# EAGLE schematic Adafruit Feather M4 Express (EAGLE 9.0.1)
COMPANY: ADAFRUIT INDUSTRIES; DRAWN: KTOWN; REV: B
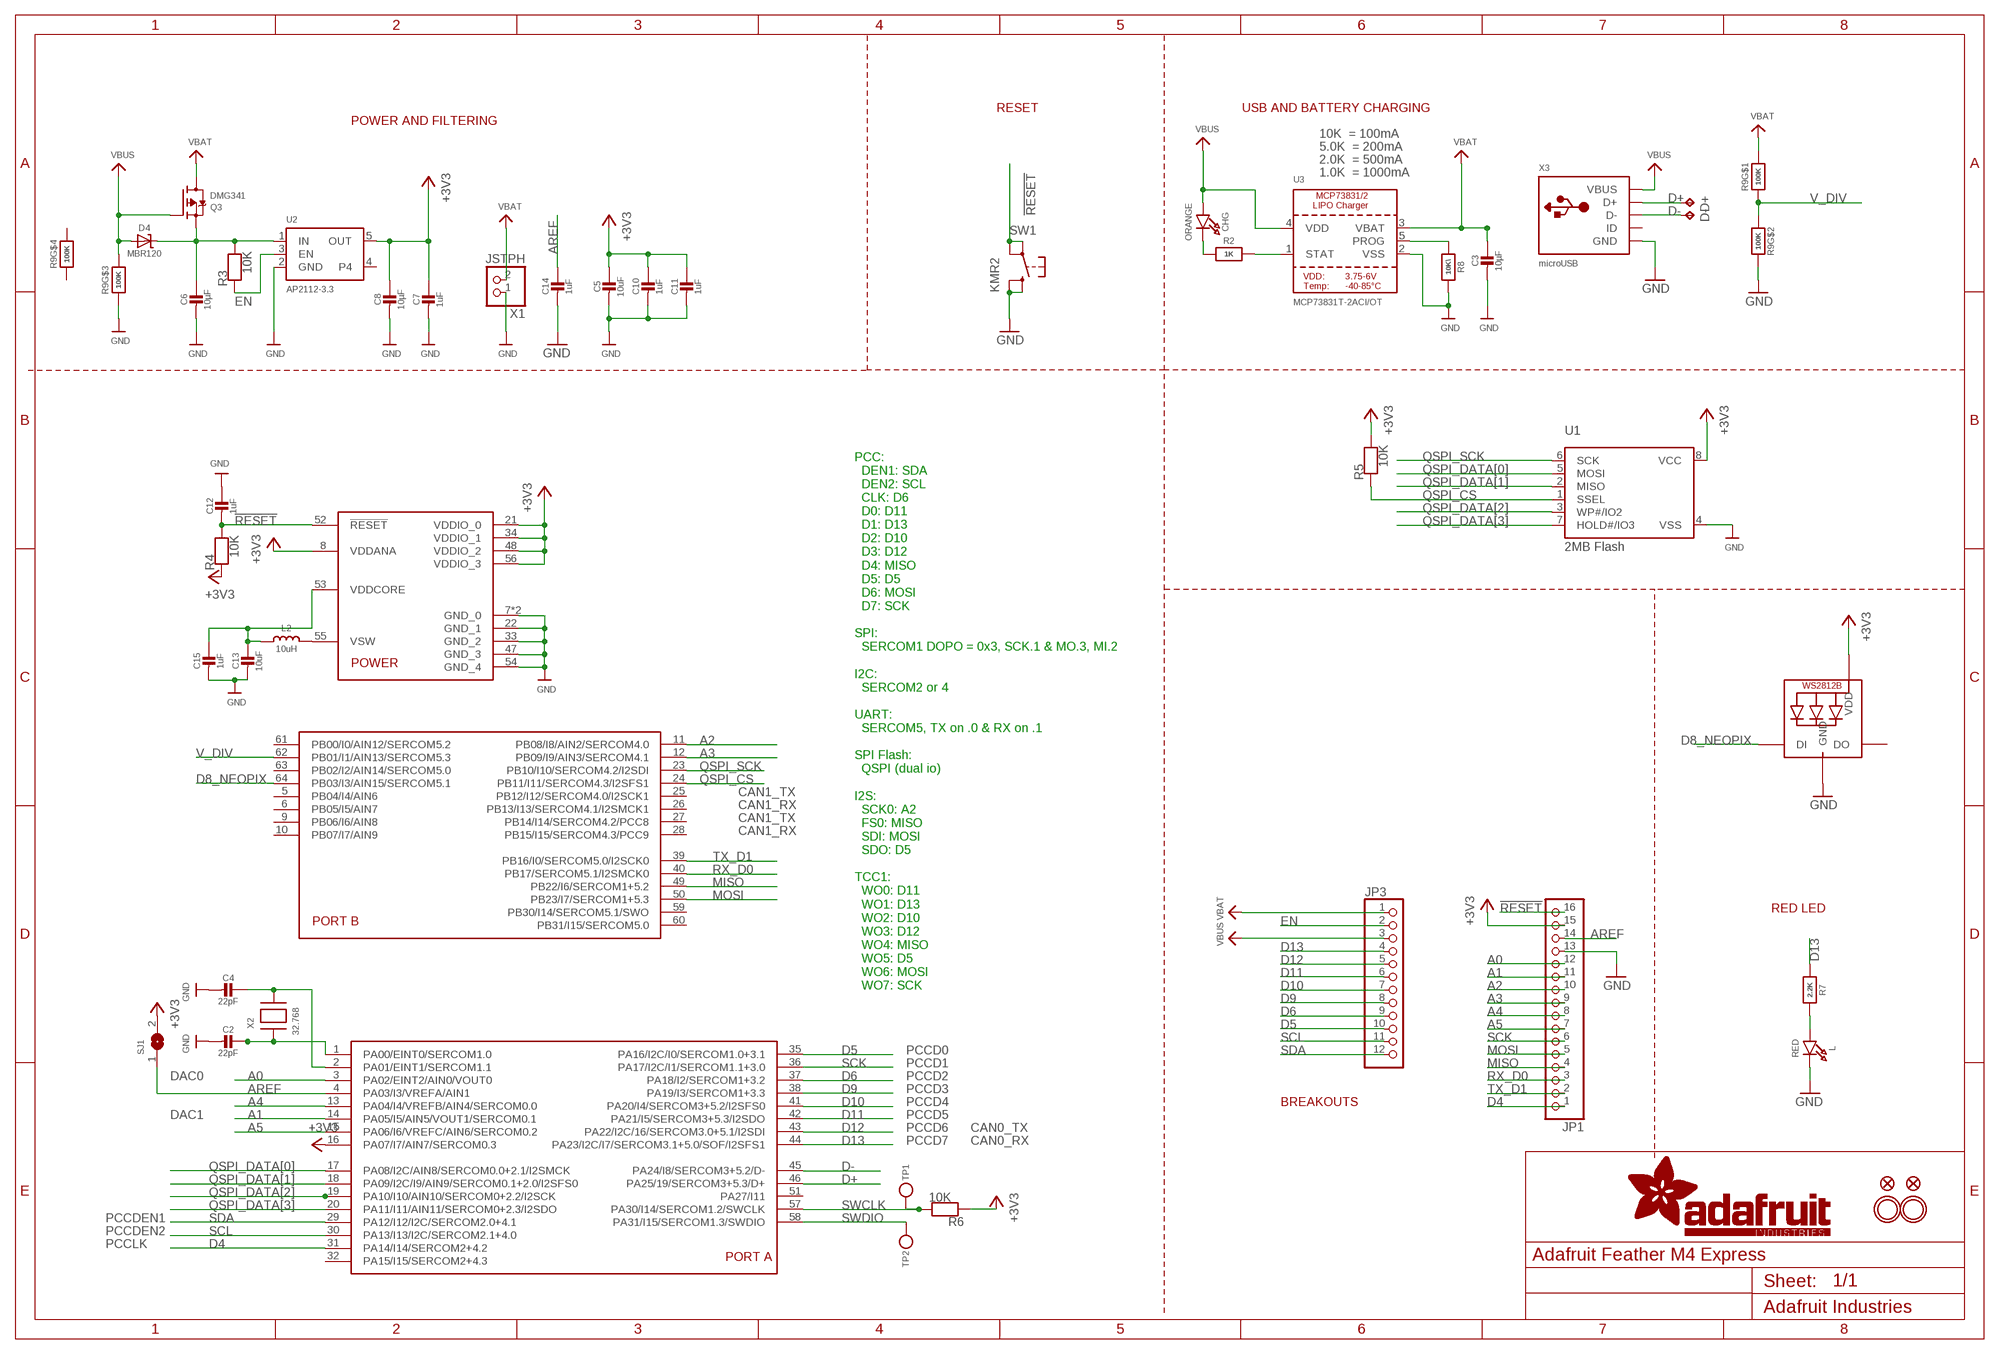
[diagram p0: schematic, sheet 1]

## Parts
C2  22pF  CAP_CERAMIC0603_NO  [0603-NO]
C3  10µF  CAP_CERAMIC0805-NOOUTLINE  [0805-NO]
C4  22pF  CAP_CERAMIC0603_NO  [0603-NO]
C5  10uF  CAP_CERAMIC0805-NOOUTLINE  [0805-NO]
C6  10µF  CAP_CERAMIC0805-NOOUTLINE  [0805-NO]
C7  1uF  CAP_CERAMIC0603_NO  [0603-NO]
C8  10µF  CAP_CERAMIC0805-NOOUTLINE  [0805-NO]
C10  1uF  CAP_CERAMIC0603_NO  [0603-NO]
C11  1uF  CAP_CERAMIC0603_NO  [0603-NO]
C12  1uF  CAP_CERAMIC0603_NO  [0603-NO]
C13  10uF  CAP_CERAMIC0805-NOOUTLINE  [0805-NO]
C14  1uF  CAP_CERAMIC0603_NO  [0603-NO]
C15  1uF  CAP_CERAMIC0603_NO  [0603-NO]
CHG  ORANGE  LED0805_NOOUTLINE  [CHIPLED_0805_NOOUTLINE]
D4  MBR120  DIODE-SCHOTTKYSOD-123  [SOD-123]
D+  TPB1,27  [B1,27]
D-  TPB1,27  [B1,27]
JP1  HEADER-1X16ROUND  [1X16_ROUND]
JP3  HEADER-1X12  [1X12_ROUND]
L  RED  LED0805_NOOUTLINE  [CHIPLED_0805_NOOUTLINE]
L2  10uH  INDUCTOR  [INDUCTOR_1007]
LED1  WS2812B3535  [LED3535]
Q3  DMG341  MOSFET-P  [SOT23-R]
R2  1K  RESISTOR_0603_NOOUT  [0603-NO]
R3  10K  RESISTOR_0603_NOOUT  [0603-NO]
R4  10K  RESISTOR_0603_NOOUT  [0603-NO]
R5  10K  RESISTOR_0603_NOOUT  [0603-NO]
R6  10K  RESISTOR_0603_NOOUT  [0603-NO]
R7  2.2K  RESISTOR_0603_NOOUT  [0603-NO]
R8  10K\  RESISTOR_0603_NOOUT  [0603-NO]
R9  100K  RESISTOR_4PACK_NO  [RESPACK_4X0603_NO]
SJ1  SOLDERJUMPERCLOSED  [SOLDERJUMPER_CLOSEDWIRE]
SW1  KMR2  SWITCH_TACT_SMT4.6X2.8  [BTN_KMR2_4.6X2.8]
TP1  TESTPOINTROUND1.5MM  [TESTPOINT_ROUND_1.5MM]
TP2  TESTPOINTROUND1.5MM  [TESTPOINT_ROUND_1.5MM]
U1  2MB Flash  SPIFLASH_8PINUX  [USON8]
U2  AP2112-3.3  VREG_SOT23-5  [SOT23-5]
U3  MCP73831T-2ACI/OT  MCP73831/2  [SOT23-5]
U$14  ATSAMD51J  [PQFN64-1]
U$31  MOUNTINGHOLE2.5  [MOUNTINGHOLE_2.5_PLATED]
U$32  MOUNTINGHOLE2.5  [MOUNTINGHOLE_2.5_PLATED]
U$34  FIDUCIAL_1MM  [FIDUCIAL_1MM]
U$35  FIDUCIAL_1MM  [FIDUCIAL_1MM]
X1  JSTPH  CON_JST_PH_2PIN  [JSTPH2]
X2  32.768  XTAL-3.2X1.5  [XTAL3215]
X3  microUSB  USB_MICRO_20329_V2  [4UCONN_20329_V2]

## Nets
!RESET: C12.2 JP1.16 R4.2 SW1.A'(P1) SW1.A(P) U$14.52(!RESET)
+3V3 [power]: C5.1 C7.1 C8.1 C10.1 C11.1 JP1.15 LED1.2(VDD) R4.1 R5.2 R6.1 SJ1.2 U1.8(VCC) U2.5(OUT) U$14.8(VDDANA) U$14.16(PA07/I7/AIN7/SERCOM0.3) U$14.21(VDDIO_0) U$14.34(VDDIO_1) U$14.48(VDDIO_2) U$14.56(VDDIO_3)
A0: JP1.12 U$14.3(PA02/EINT2/AIN0/VOUT0)
A1: JP1.11 U$14.14(PA05/I5/AIN5/VOUT1/SERCOM0.1)
A2: JP1.10 U$14.11(PB08/I8/AIN2/SERCOM4.0)
A3: JP1.9 U$14.12(PB09/I9/AIN3/SERCOM4.1)
A4: JP1.8 U$14.13(PA04/I4/VREFB/AIN4/SERCOM0.0)
A5: JP1.7 U$14.15(PA06/I6/VREFC/AIN6/SERCOM0.2)
AREF: C14.1 JP1.14 SJ1.1 U$14.4(PA03/I3/VREFA/AIN1)
D4: JP1.1 U$14.31(PA14/I14/SERCOM2+4.2)
D5: JP3.10 U$14.35(PA16/I2C/I0/SERCOM1.0+3.1)
D6: JP3.9 U$14.37(PA18/I2/SERCOM1+3.2)
D8_NEOPIX: LED1.1(DI) U$14.64(PB03/I3/AIN15/SERCOM5.1)
D9: JP3.8 U$14.38(PA19/I3/SERCOM1+3.3)
D10: JP3.7 U$14.41(PA20/I4/SERCOM3+5.2/I2SFS0)
D11: JP3.6 U$14.42(PA21/I5/SERCOM3+5.3/I2SDO)
D12: JP3.5 U$14.43(PA22/I2C/16/SERCOM3.0+5.1/I2SDI)
D13: JP3.4 R7.1 U$14.44(PA23/I2C/I7/SERCOM3.1+5.0/SOF/I2SFS1)
D+: D+.TP U$14.46(PA25/19/SERCOM3+5.3/D+) X3.D+
D-: D-.TP U$14.45(PA24/I8/SERCOM3+5.2/D-) X3.D-
EN: JP3.2 R3.1 U2.3(EN)
GND [gnd]: C2.2 C3.2 C4.2 C5.2 C6.2 C7.2 C8.2 C10.2 C11.2 C12.1 C13.2 C14.2 C15.2 JP1.13 L.C LED1.4(GND) R8.2 R9.3 R9.7 SW1.B'(S1) SW1.B(S) U1.4(VSS) U2.2(GND) U3.2(VSS) U$14.7(GND_0) U$14.22(GND_1) U$14.33(GND_2) U$14.47(GND_3) U$14.54(GND_4) U$14.EXP(GND_0) X1.1 X3.BASE@1(GND) X3.BASE@2(GND) X3.GND X3.SPRT@1(GND) X3.SPRT@2(GND) X3.SPRT@3(GND) X3.SPRT@4(GND)
MISO: JP1.4 U$14.49(PB22/I6/SERCOM1+5.2)
MOSI: JP1.5 U$14.50(PB23/I7/SERCOM1+5.3)
N$1: CHG.C R2.1
N$2: L.A R7.2
N$3: R2.2 U3.1(STAT)
N$4: R8.1 U3.5(PROG)
N$5: C2.1 U$14.1(PA00/EINT0/SERCOM1.0) X2.P$1
N$7: C4.1 U$14.2(PA01/EINT1/SERCOM1.1) X2.P$2
N$11: L2.P$2 U$14.55(VSW)
QSPI_CS: R5.1 U1.1(SSEL) U$14.24(PB11/I11/SERCOM4.3/I2SFS1)
QSPI_DATA[0]: U1.5(MOSI) U$14.17(PA08/I2C/AIN8/SERCOM0.0+2.1/I2SMCK)
QSPI_DATA[1]: U1.2(MISO) U$14.18(PA09/I2C/I9/AIN9/SERCOM0.1+2.0/I2SFS0)
QSPI_DATA[2]: U1.3(WP#/IO2) U$14.19(PA10/I10/AIN10/SERCOM0+2.2/I2SCK)
QSPI_DATA[3]: U1.7(HOLD#/IO3) U$14.20(PA11/I11/AIN11/SERCOM0+2.3/I2SDO)
QSPI_SCK: U1.6(SCK) U$14.23(PB10/I10/SERCOM4.2/I2SDI)
RX_D0: JP1.3 U$14.40(PB17/SERCOM5.1/I2SMCK0)
SCK: JP1.6 U$14.36(PA17/I2C/I1/SERCOM1.1+3.0)
SCL: JP3.11 U$14.30(PA13/I13/I2C/SERCOM2.1+4.0)
SDA: JP3.12 U$14.29(PA12/I12/I2C/SERCOM2.0+4.1)
SWCLK: R6.2 TP1.P$1 U$14.57(PA30/I14/SERCOM1.2/SWCLK)
SWDIO: TP2.P$1 U$14.58(PA31/I15/SERCOM1.3/SWDIO)
TX_D1: JP1.2 U$14.39(PB16/I0/SERCOM5.0/I2SCK0)
V_DIV: R9.1 R9.2 U$14.62(PB01/I1/AIN13/SERCOM5.3)
VBAT [power]: C3.1 JP3.1 Q3.3(D) R9.8 U3.3(VBAT) X1.2
VBUS [power]: CHG.A D4.A JP3.3 Q3.1(G) R9.6 U3.4(VDD) X3.VBUS
VDDCORE1: C13.1 C15.1 L2.P$1 U$14.53(VDDCORE)
VHI: C6.1 D4.C Q3.2(S) R3.2 U2.1(IN)
Unconnected: LED1.3(DO) R9.4 R9.5 U2.4 U$14.5(PB04/I4/AIN6) U$14.6(PB05/I5/AIN7) U$14.9(PB06/I6/AIN8) U$14.10(PB07/I7/AIN9) U$14.25(PB12/I12/SERCOM4.0/I2SCK1) U$14.26(PB13/I13/SERCOM4.1/I2SMCK1) U$14.27(PB14/I14/SERCOM4.2/PCC8) U$14.28(PB15/I15/SERCOM4.3/PCC9) U$14.32(PA15/I15/SERCOM2+4.3) U$14.51(PA27/I11) U$14.59(PB30/I14/SERCOM5.1/SWO) U$14.60(PB31/I15/SERCOM5.0) U$14.61(PB00/I0/AIN12/SERCOM5.2) U$14.63(PB02/I2/AIN14/SERCOM5.0) X3.ID

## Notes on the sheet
- RESET | USB AND BATTERY CHARGING
- POWER AND FILTERING
- 10K  = 100mA
- 5.0K  = 200mA
- 2.0K  = 500mA
- 1.0K  = 1000mA
- CAN1_TX
- CAN1_RX
- CAN1_TX
- CAN1_RX
- RED LED
- PCC:
    DEN1: SDA
    DEN2: SCL
    CLK: D6
    D0: D11
    D1: D13
    D2: D10
    D3: D12
    D4: MISO
    D5: D5
    D6: MOSI
    D7: SCK
  
  SPI:
    SERCOM1 DOPO = 0x3, SCK.1 & MO.3, MI.2
  
  I2C:
    SERCOM2 or 4
  
  UART:
    SERCOM5, TX on .0 & RX on .1
  
  SPI Flash:
    QSPI (dual io)
  
  I2S:
    SCK0: A2
    FS0: MISO
    SDI: MOSI
    SDO: D5
  
  TCC1:
    WO0: D11
    WO1: D13
    WO2: D10
    WO3: D12
    WO4: MISO
    WO5: D5
    WO6: MOSI
    WO7: SCK
- PCCD0
- PCCD1
- DAC0 | PCCD2
- PCCD3
- PCCD4 | BREAKOUTS
- DAC1 | PCCD5
- PCCD6 | CAN0_TX
- PCCD7 | CAN0_RX
- PCCDEN1
- PCCDEN2
- PCCLK

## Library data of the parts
C2-C8 C10-C15 = microbuilder:CAP_CERAMIC: Ceramic Capacitors
CHG L = microbuilder:LED: LED
D4 = microbuilder:DIODE-SCHOTTKY
D+ D- = testpad:TP: Test pad
JP1 = microbuilder:HEADER-1X16: PIN HEADER
JP3 = microbuilder:HEADER-1X12
L2 = microbuilder:INDUCTOR: Inductors
LED1 = microbuilder:WS2812B
Q3 = microbuilder:MOSFET-P: P-Channel Mosfet LEGEND VDS: Voltage Drain-Source ID: Drain Current RDS(ON): Drain-Source On-State Resistance VGS(TH): Gate-Source Threshold Voltage CISS: Drain-Source Input Capacitance SOT-23 Name VDS ID RDS(ON) VGS(TH) CISS Order Number IRLML5103 30V 760mA 600 mOhm -- 75pF @ 25V Digikey: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
R2-R8 = microbuilder:RESISTOR: Resistors
R9 = microbuilder:RESISTOR_4PACK: Resistor Packs (4 resistors) 4 x 0603 10K 1/16W - Digikey: YC164J-10KCT-ND
SJ1 = microbuilder:SOLDERJUMPER: SMD Solder JUMPER
SW1 = microbuilder:SWITCH_TACT_SMT: SMT Tact Switches 6x6mm - Digikey: P12940SCT-ND KMR2 (4.6x2.8mm) - Digikey: 401-1426-1-ND EVQ-PQHB55 - Light Touch, 160GF (4.5x4.5mm) - Digikey: P8090SCT-ND KMT0 - KMT021 NGJ LHS (etc.) IP68/Waterproof - Digikey: CKN10289CT-ND
TP1 TP2 = microbuilder:TESTPOINT: Test Point
U1 = microbuilder:SPIFLASH_8PIN: SOIC8 SPI Flash Be careful with the size since SOIC8 flash comes in several 'widths' SOIC8 150 mil M25P16 - 16Mbit (2Mbit x 8) Serial Flash (75MHz SPI Bus), Supply: 2.7-3.6V Digikey: SOIC8 - M25P16-VMN6P-ND SOIC8 208 mil W25Q16BVSSIG - 16Mbit (2Mbit x 8) Serial Flash (104MHz SPI Bus), Supply: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
U2 = microbuilder:VREG_SOT23-5: SOT23-5 Fixed Voltage Regulators Part Current Out V Out V In V Dropout θJA (°C/W) TJ (°C) Digikey Part No. ADP121 150mA 3.3V 3.4-5.5V 0.09V @ 150mA -- -- ADP121-AUJZ33R7CT-ND ADP121 150mA 3.0V 3.1-5.5V 0.09V @ 150mA -- -- ADP121-AUJZ30R7CT-ND ADP122 300mA 3.3V 3.4-5.5V 0.085V @ 300mA -- --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
U3 = microbuilder:MCP73831/2: MCP73831/2 LIPO Charger VDD: 3.75 - 6V Temp -40 - 85°C Programmable Charge Rate: 15-500mA NOTE: STAT is a tri-state logic output on the MCP73831 and an open-drain output on the MCP73832. SOT23-5 with 4.2V output and tri-state logic on STAT = MCP73831T-2ACI/OT
U$14 = microbuilder:ATSAMD51J: ATSAMD51J cortex m4 microcontroller
U$31 U$32 = microbuilder:MOUNTINGHOLE: Mounting Hole; BOM: EXCLUDE
U$34 U$35 = microbuilder:FIDUCIAL: Fiducial Alignment Points; BOM: EXCLUDE
X1 = microbuilder:CON_JST_PH_2PIN: JST 2-Pin Right-Angle Connector
X2 = adafruit2:XTAL: Low cost SMT crystals, no capacitors included
X3 = microbuilder:USB: USB Connectors USBMINIB - Surface Mount Female Mini-B USB Connector 4UConnector: 06564

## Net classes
1 power: width 0.305 mm
2 gnd: width 0.254 mm

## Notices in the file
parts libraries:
microbuilder: This work is placed in the public domain, and may be freely used for commercial and non-commercial work with the following conditions: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
